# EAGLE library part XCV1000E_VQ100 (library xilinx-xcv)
xcv1000e_vq100 edit this description Auto generated by make-symbol-device-package-bsdl.ulp Rev. 26 Source: xcv1000e_vq100.bsd
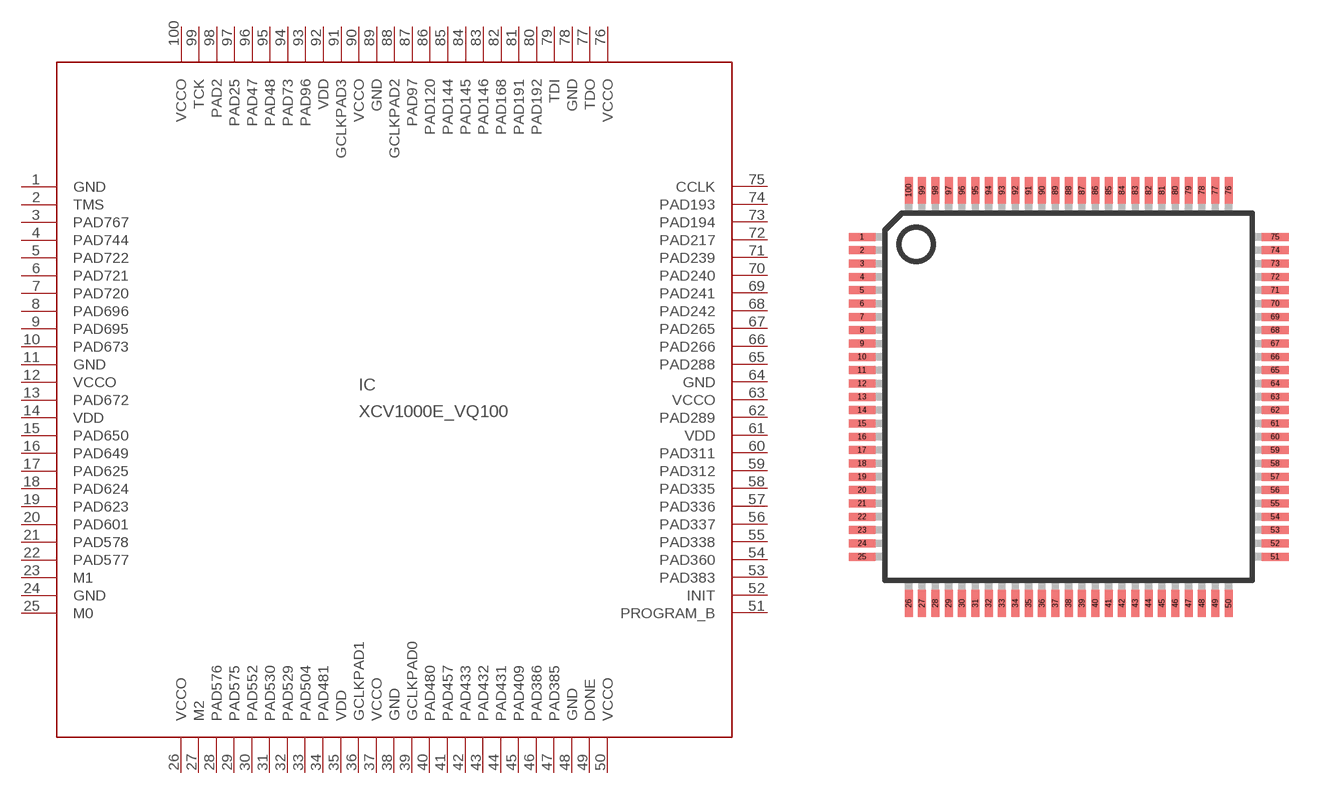
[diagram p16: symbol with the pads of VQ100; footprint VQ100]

Designator prefix IC

## XCV1000E_VQ100 (OC_FARNELL: unknown; OC_NEWARK: unknown)  [VQ100]
1  GND  pwr
2  TMS  in
3  PAD767
4  PAD744
5  PAD722
6  PAD721
7  PAD720
8  PAD696
9  PAD695
10  PAD673
11  GND  pwr
12  VCCO  pwr
13  PAD672
14  VDD  pwr
15  PAD650
16  PAD649
17  PAD625
18  PAD624
19  PAD623
20  PAD601
21  PAD578
22  PAD577
23  M1  in
24  GND  pwr
25  M0  in
26  VCCO  pwr
27  M2  in
28  PAD576
29  PAD575
30  PAD552
31  PAD530
32  PAD529
33  PAD504
34  PAD481
35  VDD  pwr
36  GCLKPAD1  in
37  VCCO  pwr
38  GND  pwr
39  GCLKPAD0  in
40  PAD480
41  PAD457
42  PAD433
43  PAD432
44  PAD431
45  PAD409
46  PAD386
47  PAD385
48  GND  pwr
49  DONE
50  VCCO  pwr
51  PROGRAM_B  in
52  INIT
53  PAD383
54  PAD360
55  PAD338
56  PAD337
57  PAD336
58  PAD335
59  PAD312
60  PAD311
61  VDD  pwr
62  PAD289
63  VCCO  pwr
64  GND  pwr
65  PAD288
66  PAD266
67  PAD265
68  PAD242
69  PAD241
70  PAD240
71  PAD239
72  PAD217
73  PAD194
74  PAD193
75  CCLK
76  VCCO  pwr
77  TDO  out
78  GND  pwr
79  TDI  in
80  PAD192
81  PAD191
82  PAD168
83  PAD146
84  PAD145
85  PAD144
86  PAD120
87  PAD97
88  GCLKPAD2  in
89  GND  pwr
90  VCCO  pwr
91  GCLKPAD3  in
92  VDD  pwr
93  PAD96
94  PAD73
95  PAD48
96  PAD47
97  PAD25
98  PAD2
99  TCK  in
100  VCCO  pwr

## Footprint VQ100 (pad centres in mm)
VQ100 Auto generated by make-symbol-device-package-bsdl.ulp Rev. 26
smd 1 x 0.3: 1 -7.75,6; 2 -7.75,5.5; 3 -7.75,5; 4 -7.75,4.5; 5 -7.75,4; 6 -7.75,3.5; 7 -7.75,3; 8 -7.75,2.5; 9 -7.75,2; 10 -7.75,1.5; 11 -7.75,1; 12 -7.75,0.5; 13 -7.75,0; 14 -7.75,-0.5; 15 -7.75,-1; 16 -7.75,-1.5; 17 -7.75,-2; 18 -7.75,-2.5; 19 -7.75,-3; 20 -7.75,-3.5; 21 -7.75,-4; 22 -7.75,-4.5; 23 -7.75,-5; 24 -7.75,-5.5; 25 -7.75,-6; 51 7.75,-6; 52 7.75,-5.5; 53 7.75,-5; 54 7.75,-4.5; 55 7.75,-4; 56 7.75,-3.5; 57 7.75,-3; 58 7.75,-2.5; 59 7.75,-2; 60 7.75,-1.5; 61 7.75,-1; 62 7.75,-0.5; 63 7.75,0; 64 7.75,0.5; 65 7.75,1; 66 7.75,1.5; 67 7.75,2; 68 7.75,2.5; 69 7.75,3; 70 7.75,3.5; 71 7.75,4; 72 7.75,4.5; 73 7.75,5; 74 7.75,5.5; 75 7.75,6
smd 0.3 x 1: 26 -6,-7.75; 27 -5.5,-7.75; 28 -5,-7.75; 29 -4.5,-7.75; 30 -4,-7.75; 31 -3.5,-7.75; 32 -3,-7.75; 33 -2.5,-7.75; 34 -2,-7.75; 35 -1.5,-7.75; 36 -1,-7.75; 37 -0.5,-7.75; 38 0,-7.75; 39 0.5,-7.75; 40 1,-7.75; 41 1.5,-7.75; 42 2,-7.75; 43 2.5,-7.75; 44 3,-7.75; 45 3.5,-7.75; 46 4,-7.75; 47 4.5,-7.75; 48 5,-7.75; 49 5.5,-7.75; 50 6,-7.75; 76 6,7.75; 77 5.5,7.75; 78 5,7.75; 79 4.5,7.75; 80 4,7.75; 81 3.5,7.75; 82 3,7.75; 83 2.5,7.75; 84 2,7.75; 85 1.5,7.75; 86 1,7.75; 87 0.5,7.75; 88 0,7.75; 89 -0.5,7.75; 90 -1,7.75; 91 -1.5,7.75; 92 -2,7.75; 93 -2.5,7.75; 94 -3,7.75; 95 -3.5,7.75; 96 -4,7.75; 97 -4.5,7.75; 98 -5,7.75; 99 -5.5,7.75; 100 -6,7.75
